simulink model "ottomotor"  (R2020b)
settings: Solver=ode45  StartTime=0.0  StopTime=0.1  FixedStep=0.01  RelTol=1e-6  AbsTol=1e-10
model workspace (MAT data in the model file):
  Pe = 0.65
  Qges = 91
  R = 287
  TW = 300
  Vc = 5.15e-06
  a = 6.91
  alphaW = 350
  be = 400
  cp = 1050
  d = 0.039
  dphiB = 1.04716666667
  e = 8
  h = 0.029
  l = 0.052
  lam = 0.25
  m = 2
  mL = 3.95e-05
  n = 3350
  r = 0.013

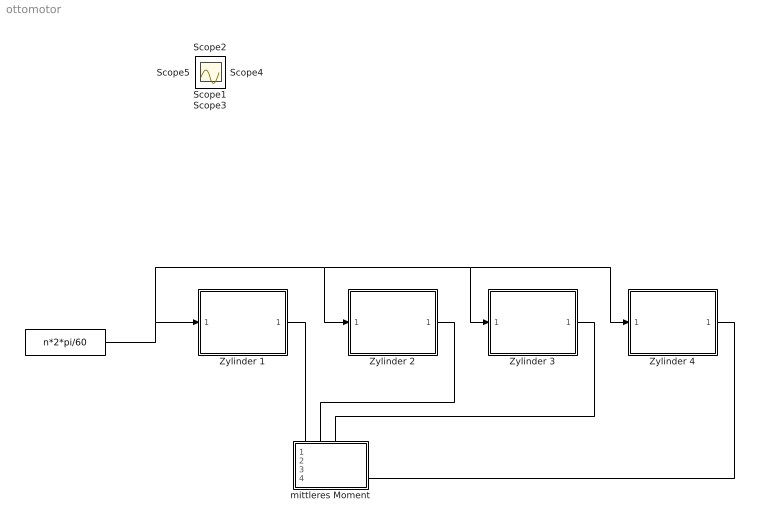
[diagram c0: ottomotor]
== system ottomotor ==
  "  " : Constant  Value=n*2*pi/60
  Zylinder 1 : Subsystem
  Zylinder 2 : Subsystem
  Zylinder 3 : Subsystem
  Zylinder 4 : Subsystem
  mittleres Moment : Subsystem
  Scope{1..5} (5 alike) : Scope
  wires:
  "  "/1 -> Zylinder 1/1(In2), Zylinder 4/1(In2), Zylinder 3/1(In2), Zylinder 2/1(In2)
  Zylinder 4/1(Md4) -> mittleres Moment/4(Md4)
  Zylinder 3/1(Md3) -> mittleres Moment/3(Md3)
  Zylinder 1/1(Md1) -> mittleres Moment/1(Md1)
  Zylinder 2/1(Md2) -> mittleres Moment/2(Md2)

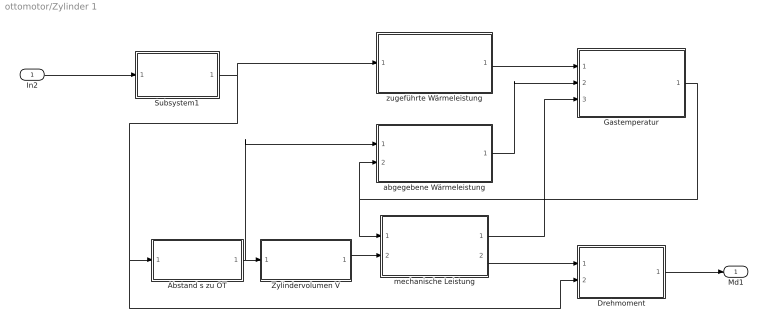
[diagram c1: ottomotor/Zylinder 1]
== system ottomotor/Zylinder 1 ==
  In2 : Inport
  Abstand s zu OT : Subsystem
  Drehmoment : Subsystem
  Gastemperatur : Subsystem
  Subsystem1 : Subsystem
  Zylindervolumen V : Subsystem
  abgegebene Wärmeleistung : Subsystem
  mechanische Leistung : Subsystem
  zugeführte Wärmeleistung : Subsystem
  Md1 : Outport
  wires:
  Gastemperatur/1(T) -> mechanische Leistung/1(T), abgegebene Wärmeleistung/2(T)
  abgegebene Wärmeleistung/1(Q_dot_ab) -> Gastemperatur/2(Q_dot_ab)
  In2/1 -> Subsystem1/1(In2)
  mechanische Leistung/1(W_dot) -> Gastemperatur/3(W_dot)
  Zylindervolumen V/1(V) -> mechanische Leistung/2(V)
  Abstand s zu OT/1(s) -> abgegebene Wärmeleistung/1(s), Zylindervolumen V/1(In1)
  zugeführte Wärmeleistung/1(Q_dot_zu) -> Gastemperatur/1(Q_dot_zu)
  mechanische Leistung/2(pz) -> Drehmoment/1(pz)
  Subsystem1/1(phi) -> Drehmoment/2(phi), Abstand s zu OT/1(phi), zugeführte Wärmeleistung/1(phi)
  Drehmoment/1(Md) -> Md1/1

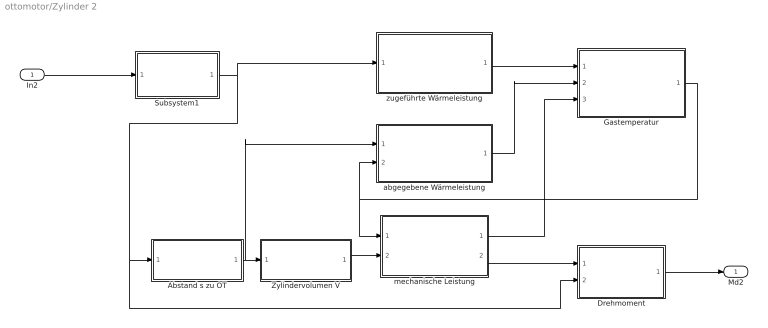
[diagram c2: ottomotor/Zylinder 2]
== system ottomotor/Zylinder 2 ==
  In2 : Inport
  Abstand s zu OT : Subsystem
  Drehmoment : Subsystem
  Gastemperatur : Subsystem
  Subsystem1 : Subsystem
  Zylindervolumen V : Subsystem
  abgegebene Wärmeleistung : Subsystem
  mechanische Leistung : Subsystem
  zugeführte Wärmeleistung : Subsystem
  Md2 : Outport
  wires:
  Gastemperatur/1(T) -> mechanische Leistung/1(T), abgegebene Wärmeleistung/2(T)
  abgegebene Wärmeleistung/1(Q_dot_ab) -> Gastemperatur/2(Q_dot_ab)
  In2/1 -> Subsystem1/1(In2)
  mechanische Leistung/1(W_dot) -> Gastemperatur/3(W_dot)
  Zylindervolumen V/1(V) -> mechanische Leistung/2(V)
  Abstand s zu OT/1(s) -> abgegebene Wärmeleistung/1(s), Zylindervolumen V/1(In1)
  zugeführte Wärmeleistung/1(Q_dot_zu) -> Gastemperatur/1(Q_dot_zu)
  mechanische Leistung/2(pz) -> Drehmoment/1(pz)
  Subsystem1/1(phi) -> Drehmoment/2(phi), Abstand s zu OT/1(phi), zugeführte Wärmeleistung/1(phi)
  Drehmoment/1(Md) -> Md2/1

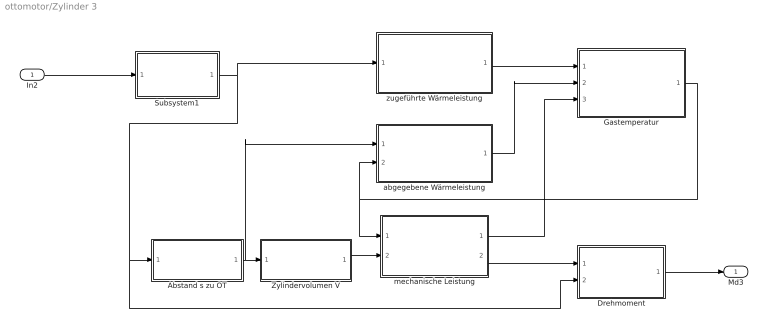
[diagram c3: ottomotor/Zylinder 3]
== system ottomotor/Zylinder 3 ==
  In2 : Inport
  Abstand s zu OT : Subsystem
  Drehmoment : Subsystem
  Gastemperatur : Subsystem
  Subsystem1 : Subsystem
  Zylindervolumen V : Subsystem
  abgegebene Wärmeleistung : Subsystem
  mechanische Leistung : Subsystem
  zugeführte Wärmeleistung : Subsystem
  Md3 : Outport
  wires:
  mechanische Leistung/2(pz) -> Drehmoment/1(pz)
  Abstand s zu OT/1(s) -> abgegebene Wärmeleistung/1(s), Zylindervolumen V/1(In1)
  Drehmoment/1(Md) -> Md3/1
  In2/1 -> Subsystem1/1(In2)
  mechanische Leistung/1(W_dot) -> Gastemperatur/3(W_dot)
  Zylindervolumen V/1(V) -> mechanische Leistung/2(V)
  abgegebene Wärmeleistung/1(Q_dot_ab) -> Gastemperatur/2(Q_dot_ab)
  Gastemperatur/1(T) -> mechanische Leistung/1(T), abgegebene Wärmeleistung/2(T)
  Subsystem1/1(phi) -> Drehmoment/2(phi), Abstand s zu OT/1(phi), zugeführte Wärmeleistung/1(phi)
  zugeführte Wärmeleistung/1(Q_dot_zu) -> Gastemperatur/1(Q_dot_zu)

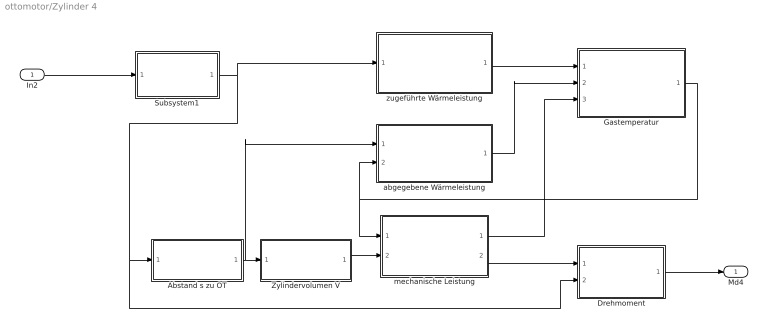
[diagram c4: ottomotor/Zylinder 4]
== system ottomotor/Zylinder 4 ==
  In2 : Inport
  Abstand s zu OT : Subsystem
  Drehmoment : Subsystem
  Gastemperatur : Subsystem
  Subsystem1 : Subsystem
  Zylindervolumen V : Subsystem
  abgegebene Wärmeleistung : Subsystem
  mechanische Leistung : Subsystem
  zugeführte Wärmeleistung : Subsystem
  Md4 : Outport
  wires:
  Gastemperatur/1(T) -> mechanische Leistung/1(T), abgegebene Wärmeleistung/2(T)
  Zylindervolumen V/1(V) -> mechanische Leistung/2(V)
  mechanische Leistung/1(W_dot) -> Gastemperatur/3(W_dot)
  Subsystem1/1(phi) -> Drehmoment/2(phi), Abstand s zu OT/1(phi), zugeführte Wärmeleistung/1(phi)
  zugeführte Wärmeleistung/1(Q_dot_zu) -> Gastemperatur/1(Q_dot_zu)
  abgegebene Wärmeleistung/1(Q_dot_ab) -> Gastemperatur/2(Q_dot_ab)
  Abstand s zu OT/1(s) -> abgegebene Wärmeleistung/1(s), Zylindervolumen V/1(In1)
  mechanische Leistung/2(pz) -> Drehmoment/1(pz)
  Drehmoment/1(Md) -> Md4/1
  In2/1 -> Subsystem1/1(In2)

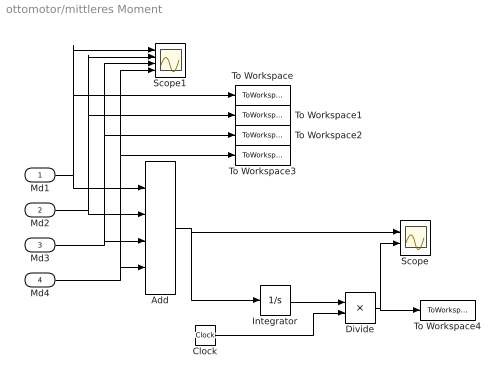
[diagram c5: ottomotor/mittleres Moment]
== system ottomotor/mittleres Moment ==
  Md1 : Inport
  Md2 : Inport  Port=2
  Md3 : Inport  Port=3
  Md4 : Inport  Port=4
  Add : Sum  Inputs=++++
  Clock : Clock
  Divide : Product  Inputs=*/
  Integrator : Integrator
  Scope : Scope  NumInputPorts=2
  Scope1 : Scope  NumInputPorts=4
  To Workspace : ToWorkspace  VariableName=Md1  SaveFormat=Timeseries  SampleTime=-1
  To Workspace1 : ToWorkspace  VariableName=Md2  SaveFormat=Timeseries  SampleTime=-1
  To Workspace2 : ToWorkspace  VariableName=Md3  SaveFormat=Timeseries  SampleTime=-1
  To Workspace3 : ToWorkspace  VariableName=Md4  SaveFormat=Timeseries  SampleTime=-1
  To Workspace4 : ToWorkspace  VariableName=Mdm  SaveFormat=Timeseries  SampleTime=-1
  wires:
  Md1/1 -> To Workspace/1, Scope1/1, Add/1
  Md2/1 -> To Workspace1/1, Scope1/2, Add/2
  Md4/1 -> Scope1/4, To Workspace3/1, Add/4
  Add/1 -> Integrator/1, Scope/1
  Integrator/1 -> Divide/1
  Clock/1 -> Divide/2
  Divide/1 -> To Workspace4/1, Scope/2
  Md3/1 -> Scope1/3, To Workspace2/1, Add/3

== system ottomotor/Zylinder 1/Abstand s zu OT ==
  phi : Inport
  Abstand s zu OT : Fcn  Expr=r+l-r*(cos(u)+1/lam-lam/4+lam/4*cos(2*u))
  Scope : Scope
  s : Outport
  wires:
  phi/1 -> Abstand s zu OT/1
  Abstand s zu OT/1 -> Scope/1, s/1

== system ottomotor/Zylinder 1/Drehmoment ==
  pz : Inport
  phi : Inport  Port=2
  Faktor : Fcn  Expr=sin(u)+lam*sin(2*u)/(2*sqrt(1-lam^2*sin(u)^2))
  Gain : Gain  Gain=r
  Kolbenkraft Fk : Fcn  Expr=d^2/4*pi*u
  Product : Product
  Scope : Scope
  Md : Outport
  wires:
  pz/1 -> Kolbenkraft Fk/1
  phi/1 -> Faktor/1
  Kolbenkraft Fk/1 -> Gain/1
  Gain/1 -> Product/1
  Faktor/1 -> Product/2
  Product/1 -> Scope/1, Md/1

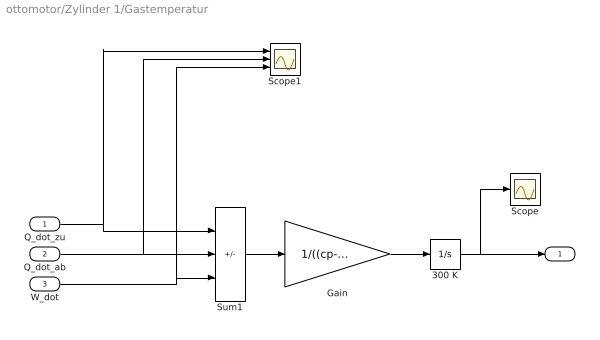
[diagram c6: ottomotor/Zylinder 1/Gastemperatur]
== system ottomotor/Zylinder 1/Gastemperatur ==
  Q_dot_zu : Inport
  Q_dot_ab : Inport  Port=2
  W_dot : Inport  Port=3
  300 K : Integrator  InitialCondition=300
  Gain : Gain  Gain=1/((cp-R)*mL)  SaturateOnIntegerOverflow=on
  Scope : Scope
  Scope1 : Scope  NumInputPorts=3
  Sum1 : Sum  Inputs=+--  SaturateOnIntegerOverflow=on
  T : Outport
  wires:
  Sum1/1 -> Gain/1
  W_dot/1 -> Scope1/3, Sum1/3
  Gain/1 -> 300 K/1
  Q_dot_zu/1 -> Scope1/1, Sum1/1
  Q_dot_ab/1 -> Scope1/2, Sum1/2
  300 K/1 -> Scope/1, T/1

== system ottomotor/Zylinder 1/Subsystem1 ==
  In2 : Inport
  Integrator1 : Integrator  InitialCondition=pi
  To Workspace : ToWorkspace  VariableName=phi  SaveFormat=Timeseries  SampleTime=-1
  phi : Outport
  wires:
  In2/1 -> Integrator1/1
  Integrator1/1 -> To Workspace/1, phi/1

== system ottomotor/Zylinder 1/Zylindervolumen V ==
  In1 : Inport
  Zylindervolumen V : Fcn  Expr=Vc+d^2/4*pi*u
  V : Outport
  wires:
  In1/1 -> Zylindervolumen V/1
  Zylindervolumen V/1 -> V/1

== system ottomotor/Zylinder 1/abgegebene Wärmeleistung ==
  s : Inport
  T : Inport  Port=2
  Gain1 : Gain  Gain=alphaW  SaturateOnIntegerOverflow=on
  Product2 : Product  SaturateOnIntegerOverflow=on
  Sum2 : Sum  Inputs=-+|  SaturateOnIntegerOverflow=on
  Wand- temperatur : Constant  Value=TW
  wärmetauschende Oberfläche A : Fcn  Expr=2*d^2/4*pi+pi*d*u
  Q_dot_ab : Outport
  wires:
  wärmetauschende Oberfläche A/1 -> Gain1/1
  Gain1/1 -> Product2/1
  s/1 -> wärmetauschende Oberfläche A/1
  Wand- temperatur/1 -> Sum2/1
  Sum2/1 -> Product2/2
  T/1 -> Sum2/2
  Product2/1 -> Q_dot_ab/1

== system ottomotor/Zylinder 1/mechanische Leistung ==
  T : Inport
  V : Inport  Port=2
  Product3 : Product  SaturateOnIntegerOverflow=on
  Scope : Scope
  Subsystem2 : Subsystem
  dV/dt : Derivative
  W_dot : Outport
  pz : Outport  Port=2
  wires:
  T/1 -> Subsystem2/1(T)
  Subsystem2/1(pz) -> pz/1, Product3/1
  dV/dt/1 -> Product3/2
  V/1 -> dV/dt/1, Subsystem2/2(V)
  Product3/1 -> Scope/1, W_dot/1

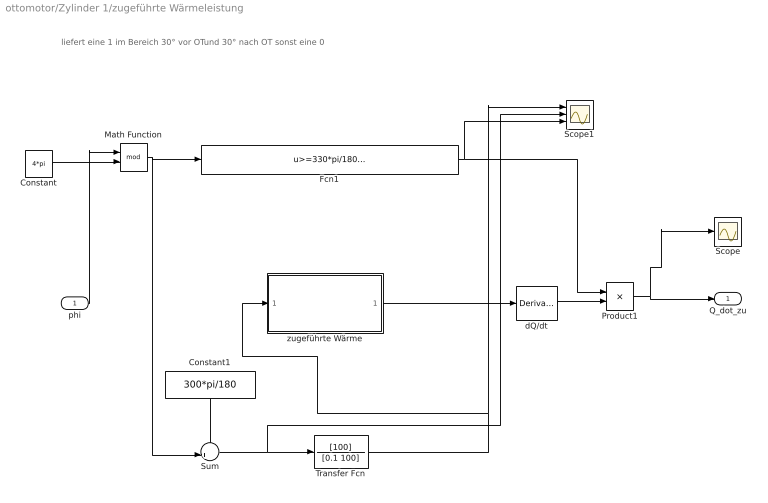
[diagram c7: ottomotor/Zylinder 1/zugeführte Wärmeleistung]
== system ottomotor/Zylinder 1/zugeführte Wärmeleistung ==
  note: liefert eine 1 im Bereich 30° vor OTund 30° nach OT sonst eine 0
  phi : Inport
  Constant : Constant  Value=4*pi
  Constant1 : Constant  Value=300*pi/180
  Fcn1 : Fcn  Expr=u>=330*pi/180 && (u<390*pi/180)
  Math Function : Math  Operator=mod
  Product1 : Product  SaturateOnIntegerOverflow=on
  Scope : Scope
  Scope1 : Scope  NumInputPorts=3
  Sum : Sum  Inputs=-+|  SaturateOnIntegerOverflow=on
  Transfer Fcn : TransferFcn  Numerator=[100]  Denominator=[0.1 100]
  dQ/dt : Derivative
  zugeführte Wärme : Subsystem
  Q_dot_zu : Outport
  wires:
  Product1/1 -> Scope/1, Q_dot_zu/1
  dQ/dt/1 -> Product1/2
  phi/1 -> Math Function/1
  Constant/1 -> Math Function/2
  Math Function/1 -> Sum/2, Fcn1/1
  Fcn1/1 -> Scope1/3, Product1/1
  Constant1/1 -> Sum/1
  Sum/1 -> Scope1/2, Transfer Fcn/1
  Transfer Fcn/1 -> zugeführte Wärme/1(phi), Scope1/1
  zugeführte Wärme/1(Q) -> dQ/dt/1

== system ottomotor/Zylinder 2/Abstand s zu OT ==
  phi : Inport
  Abstand s zu OT : Fcn  Expr=r+l-r*(cos(u)+1/lam-lam/4+lam/4*cos(2*u))
  Scope : Scope
  s : Outport
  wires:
  phi/1 -> Abstand s zu OT/1
  Abstand s zu OT/1 -> Scope/1, s/1

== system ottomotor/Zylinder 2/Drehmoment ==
  pz : Inport
  phi : Inport  Port=2
  Faktor : Fcn  Expr=sin(u)+lam*sin(2*u)/(2*sqrt(1-lam^2*sin(u)^2))
  Gain : Gain  Gain=r
  Kolbenkraft Fk : Fcn  Expr=d^2/4*pi*u
  Product : Product
  Scope : Scope
  Md : Outport
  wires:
  pz/1 -> Kolbenkraft Fk/1
  phi/1 -> Faktor/1
  Kolbenkraft Fk/1 -> Gain/1
  Gain/1 -> Product/1
  Faktor/1 -> Product/2
  Product/1 -> Scope/1, Md/1

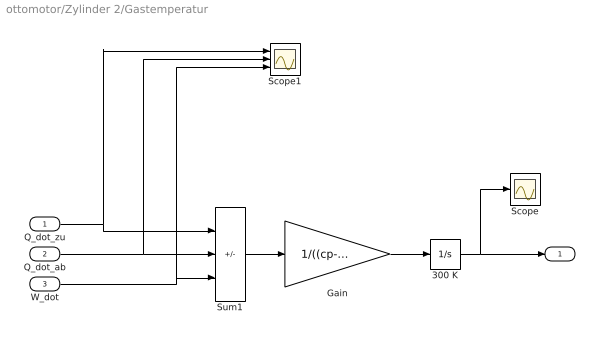
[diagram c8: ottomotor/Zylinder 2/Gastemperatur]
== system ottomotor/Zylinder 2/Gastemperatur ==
  Q_dot_zu : Inport
  Q_dot_ab : Inport  Port=2
  W_dot : Inport  Port=3
  300 K : Integrator  InitialCondition=300
  Gain : Gain  Gain=1/((cp-R)*mL)  SaturateOnIntegerOverflow=on
  Scope : Scope
  Scope1 : Scope  NumInputPorts=3
  Sum1 : Sum  Inputs=+--  SaturateOnIntegerOverflow=on
  T : Outport
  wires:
  Sum1/1 -> Gain/1
  W_dot/1 -> Scope1/3, Sum1/3
  Gain/1 -> 300 K/1
  Q_dot_zu/1 -> Scope1/1, Sum1/1
  Q_dot_ab/1 -> Scope1/2, Sum1/2
  300 K/1 -> Scope/1, T/1

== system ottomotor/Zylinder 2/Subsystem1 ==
  In2 : Inport
  Integrator1 : Integrator  InitialCondition=2*pi
  phi : Outport
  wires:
  In2/1 -> Integrator1/1
  Integrator1/1 -> phi/1

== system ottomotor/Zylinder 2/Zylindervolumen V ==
  In1 : Inport
  Zylindervolumen V : Fcn  Expr=Vc+d^2/4*pi*u
  V : Outport
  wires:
  In1/1 -> Zylindervolumen V/1
  Zylindervolumen V/1 -> V/1

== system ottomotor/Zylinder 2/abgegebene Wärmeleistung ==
  s : Inport
  T : Inport  Port=2
  Gain1 : Gain  Gain=alphaW  SaturateOnIntegerOverflow=on
  Product2 : Product  SaturateOnIntegerOverflow=on
  Sum2 : Sum  Inputs=-+|  SaturateOnIntegerOverflow=on
  Wand- temperatur : Constant  Value=TW
  wärmetauschende Oberfläche A : Fcn  Expr=2*d^2/4*pi+pi*d*u
  Q_dot_ab : Outport
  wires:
  wärmetauschende Oberfläche A/1 -> Gain1/1
  Gain1/1 -> Product2/1
  s/1 -> wärmetauschende Oberfläche A/1
  Wand- temperatur/1 -> Sum2/1
  Sum2/1 -> Product2/2
  T/1 -> Sum2/2
  Product2/1 -> Q_dot_ab/1

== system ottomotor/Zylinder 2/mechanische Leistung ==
  T : Inport
  V : Inport  Port=2
  Product3 : Product  SaturateOnIntegerOverflow=on
  Scope : Scope
  Subsystem2 : Subsystem
  dV/dt : Derivative
  W_dot : Outport
  pz : Outport  Port=2
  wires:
  T/1 -> Subsystem2/1(T)
  Subsystem2/1(pz) -> pz/1, Product3/1
  dV/dt/1 -> Product3/2
  V/1 -> dV/dt/1, Subsystem2/2(V)
  Product3/1 -> Scope/1, W_dot/1

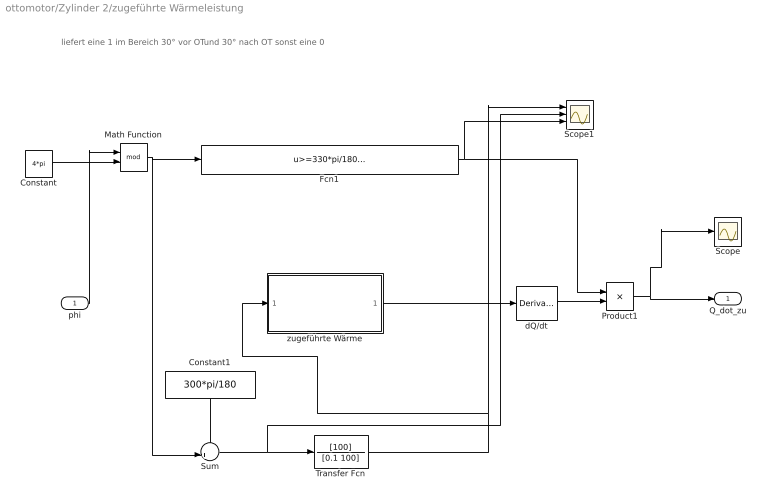
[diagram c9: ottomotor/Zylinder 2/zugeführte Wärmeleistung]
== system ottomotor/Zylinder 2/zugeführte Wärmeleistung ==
  note: liefert eine 1 im Bereich 30° vor OTund 30° nach OT sonst eine 0
  phi : Inport
  Constant : Constant  Value=4*pi
  Constant1 : Constant  Value=300*pi/180
  Fcn1 : Fcn  Expr=u>=330*pi/180 && (u<390*pi/180)
  Math Function : Math  Operator=mod
  Product1 : Product  SaturateOnIntegerOverflow=on
  Scope : Scope
  Scope1 : Scope  NumInputPorts=3
  Sum : Sum  Inputs=-+|  SaturateOnIntegerOverflow=on
  Transfer Fcn : TransferFcn  Numerator=[100]  Denominator=[0.1 100]
  dQ/dt : Derivative
  zugeführte Wärme : Subsystem
  Q_dot_zu : Outport
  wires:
  Product1/1 -> Scope/1, Q_dot_zu/1
  dQ/dt/1 -> Product1/2
  phi/1 -> Math Function/1
  Constant/1 -> Math Function/2
  Math Function/1 -> Sum/2, Fcn1/1
  Fcn1/1 -> Scope1/3, Product1/1
  Constant1/1 -> Sum/1
  Sum/1 -> Scope1/2, Transfer Fcn/1
  Transfer Fcn/1 -> zugeführte Wärme/1(phi), Scope1/1
  zugeführte Wärme/1(Q) -> dQ/dt/1

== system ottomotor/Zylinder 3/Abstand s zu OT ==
  phi : Inport
  Abstand s zu OT : Fcn  Expr=r+l-r*(cos(u)+1/lam-lam/4+lam/4*cos(2*u))
  Scope : Scope
  s : Outport
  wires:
  phi/1 -> Abstand s zu OT/1
  Abstand s zu OT/1 -> Scope/1, s/1

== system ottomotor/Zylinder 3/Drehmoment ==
  pz : Inport
  phi : Inport  Port=2
  Faktor : Fcn  Expr=sin(u)+lam*sin(2*u)/(2*sqrt(1-lam^2*sin(u)^2))
  Gain : Gain  Gain=r
  Kolbenkraft Fk : Fcn  Expr=d^2/4*pi*u
  Product : Product
  Scope : Scope
  Md : Outport
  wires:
  pz/1 -> Kolbenkraft Fk/1
  phi/1 -> Faktor/1
  Kolbenkraft Fk/1 -> Gain/1
  Gain/1 -> Product/1
  Faktor/1 -> Product/2
  Product/1 -> Scope/1, Md/1

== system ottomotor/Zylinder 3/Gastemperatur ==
  Q_dot_zu : Inport
  Q_dot_ab : Inport  Port=2
  W_dot : Inport  Port=3
  300 K : Integrator  InitialCondition=300
  Gain : Gain  Gain=1/((cp-R)*mL)  SaturateOnIntegerOverflow=on
  Scope : Scope
  Scope1 : Scope  NumInputPorts=3
  Sum1 : Sum  Inputs=+--  SaturateOnIntegerOverflow=on
  T : Outport
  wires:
  Sum1/1 -> Gain/1
  W_dot/1 -> Scope1/3, Sum1/3
  Gain/1 -> 300 K/1
  Q_dot_zu/1 -> Scope1/1, Sum1/1
  Q_dot_ab/1 -> Scope1/2, Sum1/2
  300 K/1 -> Scope/1, T/1

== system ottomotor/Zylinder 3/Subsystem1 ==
  In2 : Inport
  Integrator1 : Integrator  InitialCondition=3*pi
  phi : Outport
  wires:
  In2/1 -> Integrator1/1
  Integrator1/1 -> phi/1

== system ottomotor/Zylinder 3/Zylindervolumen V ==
  In1 : Inport
  Zylindervolumen V : Fcn  Expr=Vc+d^2/4*pi*u
  V : Outport
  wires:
  In1/1 -> Zylindervolumen V/1
  Zylindervolumen V/1 -> V/1

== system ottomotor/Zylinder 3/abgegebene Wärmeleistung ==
  s : Inport
  T : Inport  Port=2
  Gain1 : Gain  Gain=alphaW  SaturateOnIntegerOverflow=on
  Product2 : Product  SaturateOnIntegerOverflow=on
  Sum2 : Sum  Inputs=-+|  SaturateOnIntegerOverflow=on
  Wand- temperatur : Constant  Value=TW
  wärmetauschende Oberfläche A : Fcn  Expr=2*d^2/4*pi+pi*d*u
  Q_dot_ab : Outport
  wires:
  wärmetauschende Oberfläche A/1 -> Gain1/1
  Gain1/1 -> Product2/1
  s/1 -> wärmetauschende Oberfläche A/1
  Wand- temperatur/1 -> Sum2/1
  Sum2/1 -> Product2/2
  T/1 -> Sum2/2
  Product2/1 -> Q_dot_ab/1

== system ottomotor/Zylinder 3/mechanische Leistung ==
  T : Inport
  V : Inport  Port=2
  Product3 : Product  SaturateOnIntegerOverflow=on
  Scope : Scope
  Subsystem2 : Subsystem
  dV/dt : Derivative
  W_dot : Outport
  pz : Outport  Port=2
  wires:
  T/1 -> Subsystem2/1(T)
  Subsystem2/1(pz) -> pz/1, Product3/1
  dV/dt/1 -> Product3/2
  V/1 -> dV/dt/1, Subsystem2/2(V)
  Product3/1 -> Scope/1, W_dot/1

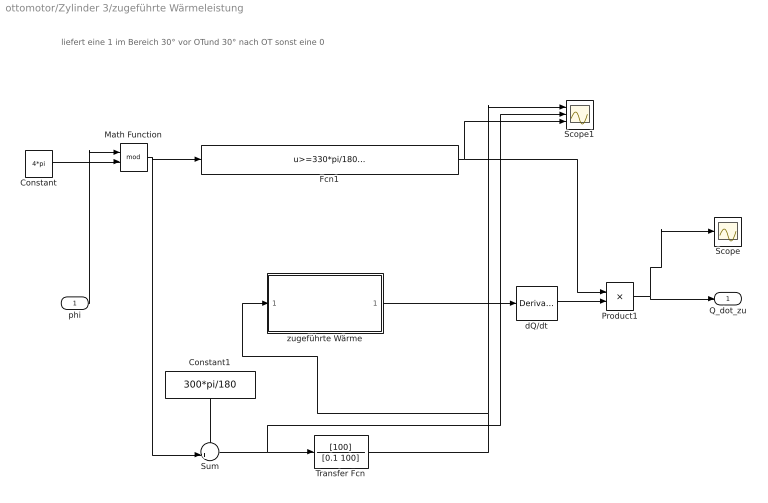
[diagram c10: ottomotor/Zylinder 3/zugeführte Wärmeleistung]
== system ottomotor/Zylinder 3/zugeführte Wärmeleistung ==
  note: liefert eine 1 im Bereich 30° vor OTund 30° nach OT sonst eine 0
  phi : Inport
  Constant : Constant  Value=4*pi
  Constant1 : Constant  Value=300*pi/180
  Fcn1 : Fcn  Expr=u>=330*pi/180 && (u<390*pi/180)
  Math Function : Math  Operator=mod
  Product1 : Product  SaturateOnIntegerOverflow=on
  Scope : Scope
  Scope1 : Scope  NumInputPorts=3
  Sum : Sum  Inputs=-+|  SaturateOnIntegerOverflow=on
  Transfer Fcn : TransferFcn  Numerator=[100]  Denominator=[0.1 100]
  dQ/dt : Derivative
  zugeführte Wärme : Subsystem
  Q_dot_zu : Outport
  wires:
  Product1/1 -> Scope/1, Q_dot_zu/1
  dQ/dt/1 -> Product1/2
  phi/1 -> Math Function/1
  Constant/1 -> Math Function/2
  Math Function/1 -> Sum/2, Fcn1/1
  Fcn1/1 -> Scope1/3, Product1/1
  Constant1/1 -> Sum/1
  Sum/1 -> Scope1/2, Transfer Fcn/1
  Transfer Fcn/1 -> zugeführte Wärme/1(phi), Scope1/1
  zugeführte Wärme/1(Q) -> dQ/dt/1

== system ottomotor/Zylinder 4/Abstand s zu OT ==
  phi : Inport
  Abstand s zu OT : Fcn  Expr=r+l-r*(cos(u)+1/lam-lam/4+lam/4*cos(2*u))
  Scope : Scope
  s : Outport
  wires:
  phi/1 -> Abstand s zu OT/1
  Abstand s zu OT/1 -> Scope/1, s/1

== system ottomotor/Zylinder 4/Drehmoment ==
  pz : Inport
  phi : Inport  Port=2
  Faktor : Fcn  Expr=sin(u)+lam*sin(2*u)/(2*sqrt(1-lam^2*sin(u)^2))
  Gain : Gain  Gain=r
  Kolbenkraft Fk : Fcn  Expr=d^2/4*pi*u
  Product : Product
  Scope : Scope
  Md : Outport
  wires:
  pz/1 -> Kolbenkraft Fk/1
  phi/1 -> Faktor/1
  Kolbenkraft Fk/1 -> Gain/1
  Gain/1 -> Product/1
  Faktor/1 -> Product/2
  Product/1 -> Scope/1, Md/1

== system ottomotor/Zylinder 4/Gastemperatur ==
  Q_dot_zu : Inport
  Q_dot_ab : Inport  Port=2
  W_dot : Inport  Port=3
  300 K : Integrator  InitialCondition=300
  Gain : Gain  Gain=1/((cp-R)*mL)  SaturateOnIntegerOverflow=on
  Scope : Scope
  Scope1 : Scope  NumInputPorts=3
  Sum1 : Sum  Inputs=+--  SaturateOnIntegerOverflow=on
  T : Outport
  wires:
  Sum1/1 -> Gain/1
  W_dot/1 -> Scope1/3, Sum1/3
  Gain/1 -> 300 K/1
  Q_dot_zu/1 -> Scope1/1, Sum1/1
  Q_dot_ab/1 -> Scope1/2, Sum1/2
  300 K/1 -> Scope/1, T/1

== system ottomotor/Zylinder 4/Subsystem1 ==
  In2 : Inport
  Integrator1 : Integrator  InitialCondition=4*pi
  phi : Outport
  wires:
  In2/1 -> Integrator1/1
  Integrator1/1 -> phi/1

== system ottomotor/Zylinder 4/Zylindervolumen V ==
  In1 : Inport
  Zylindervolumen V : Fcn  Expr=Vc+d^2/4*pi*u
  V : Outport
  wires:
  In1/1 -> Zylindervolumen V/1
  Zylindervolumen V/1 -> V/1

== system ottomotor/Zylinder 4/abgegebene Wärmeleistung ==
  s : Inport
  T : Inport  Port=2
  Gain1 : Gain  Gain=alphaW  SaturateOnIntegerOverflow=on
  Product2 : Product  SaturateOnIntegerOverflow=on
  Sum2 : Sum  Inputs=-+|  SaturateOnIntegerOverflow=on
  Wand- temperatur : Constant  Value=TW
  wärmetauschende Oberfläche A : Fcn  Expr=2*d^2/4*pi+pi*d*u
  Q_dot_ab : Outport
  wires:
  wärmetauschende Oberfläche A/1 -> Gain1/1
  Gain1/1 -> Product2/1
  s/1 -> wärmetauschende Oberfläche A/1
  Wand- temperatur/1 -> Sum2/1
  Sum2/1 -> Product2/2
  T/1 -> Sum2/2
  Product2/1 -> Q_dot_ab/1

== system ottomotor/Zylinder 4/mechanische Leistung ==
  T : Inport
  V : Inport  Port=2
  Product3 : Product  SaturateOnIntegerOverflow=on
  Scope : Scope
  Subsystem2 : Subsystem
  dV/dt : Derivative
  W_dot : Outport
  pz : Outport  Port=2
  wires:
  T/1 -> Subsystem2/1(T)
  Subsystem2/1(pz) -> pz/1, Product3/1
  dV/dt/1 -> Product3/2
  V/1 -> dV/dt/1, Subsystem2/2(V)
  Product3/1 -> Scope/1, W_dot/1

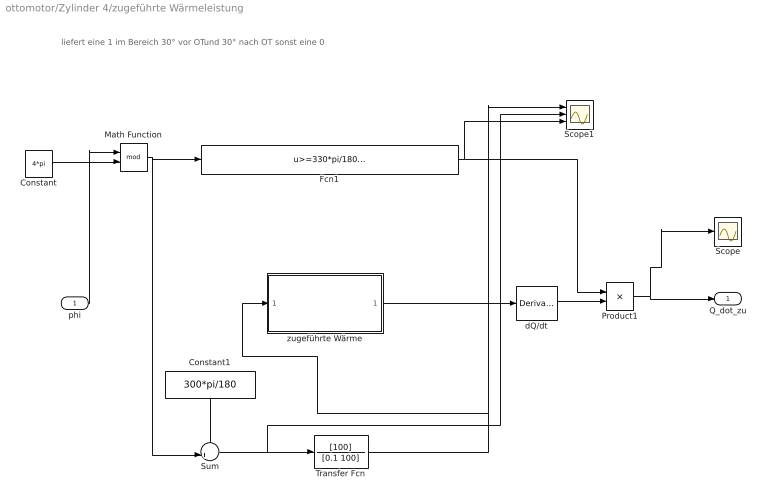
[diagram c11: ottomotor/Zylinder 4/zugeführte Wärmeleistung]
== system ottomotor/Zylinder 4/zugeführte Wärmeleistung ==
  note: liefert eine 1 im Bereich 30° vor OTund 30° nach OT sonst eine 0
  phi : Inport
  Constant : Constant  Value=4*pi
  Constant1 : Constant  Value=300*pi/180
  Fcn1 : Fcn  Expr=u>=330*pi/180 && (u<390*pi/180)
  Math Function : Math  Operator=mod
  Product1 : Product  SaturateOnIntegerOverflow=on
  Scope : Scope
  Scope1 : Scope  NumInputPorts=3
  Sum : Sum  Inputs=-+|  SaturateOnIntegerOverflow=on
  Transfer Fcn : TransferFcn  Numerator=[100]  Denominator=[0.1 100]
  dQ/dt : Derivative
  zugeführte Wärme : Subsystem
  Q_dot_zu : Outport
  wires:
  Product1/1 -> Scope/1, Q_dot_zu/1
  dQ/dt/1 -> Product1/2
  phi/1 -> Math Function/1
  Constant/1 -> Math Function/2
  Math Function/1 -> Sum/2, Fcn1/1
  Fcn1/1 -> Scope1/3, Product1/1
  Constant1/1 -> Sum/1
  Sum/1 -> Scope1/2, Transfer Fcn/1
  Transfer Fcn/1 -> zugeführte Wärme/1(phi), Scope1/1
  zugeführte Wärme/1(Q) -> dQ/dt/1

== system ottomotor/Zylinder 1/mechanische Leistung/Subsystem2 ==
  T : Inport
  V : Inport  Port=2
  Gain3 : Gain  Gain=mL*R  SaturateOnIntegerOverflow=on
  Product4 : Product  Inputs=/*  SaturateOnIntegerOverflow=on
  pz : Outport
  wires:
  V/1 -> Product4/1
  Product4/1 -> pz/1
  Gain3/1 -> Product4/2
  T/1 -> Gain3/1

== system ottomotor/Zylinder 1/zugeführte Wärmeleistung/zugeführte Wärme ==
  phi : Inport
  Fcn4 : Fcn  Expr=Qges*(1-exp(-a*(u/dphiB)^(m+1)))
  Q : Outport
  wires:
  phi/1 -> Fcn4/1
  Fcn4/1 -> Q/1

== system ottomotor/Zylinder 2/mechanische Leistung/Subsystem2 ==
  T : Inport
  V : Inport  Port=2
  Gain3 : Gain  Gain=mL*R  SaturateOnIntegerOverflow=on
  Product4 : Product  Inputs=/*  SaturateOnIntegerOverflow=on
  pz : Outport
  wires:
  V/1 -> Product4/1
  Product4/1 -> pz/1
  Gain3/1 -> Product4/2
  T/1 -> Gain3/1

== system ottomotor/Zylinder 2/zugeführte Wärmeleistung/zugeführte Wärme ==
  phi : Inport
  Fcn4 : Fcn  Expr=Qges*(1-exp(-a*(u/dphiB)^(m+1)))
  Q : Outport
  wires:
  phi/1 -> Fcn4/1
  Fcn4/1 -> Q/1

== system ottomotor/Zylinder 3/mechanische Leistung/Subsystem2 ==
  T : Inport
  V : Inport  Port=2
  Gain3 : Gain  Gain=mL*R  SaturateOnIntegerOverflow=on
  Product4 : Product  Inputs=/*  SaturateOnIntegerOverflow=on
  pz : Outport
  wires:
  V/1 -> Product4/1
  Product4/1 -> pz/1
  Gain3/1 -> Product4/2
  T/1 -> Gain3/1

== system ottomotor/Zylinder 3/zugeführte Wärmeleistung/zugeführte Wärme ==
  phi : Inport
  Fcn4 : Fcn  Expr=Qges*(1-exp(-a*(u/dphiB)^(m+1)))
  Q : Outport
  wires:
  phi/1 -> Fcn4/1
  Fcn4/1 -> Q/1

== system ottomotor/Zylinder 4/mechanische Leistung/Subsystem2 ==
  T : Inport
  V : Inport  Port=2
  Gain3 : Gain  Gain=mL*R  SaturateOnIntegerOverflow=on
  Product4 : Product  Inputs=/*  SaturateOnIntegerOverflow=on
  pz : Outport
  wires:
  V/1 -> Product4/1
  Product4/1 -> pz/1
  Gain3/1 -> Product4/2
  T/1 -> Gain3/1

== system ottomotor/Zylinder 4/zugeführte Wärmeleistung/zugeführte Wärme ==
  phi : Inport
  Fcn4 : Fcn  Expr=Qges*(1-exp(-a*(u/dphiB)^(m+1)))
  Q : Outport
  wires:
  phi/1 -> Fcn4/1
  Fcn4/1 -> Q/1
